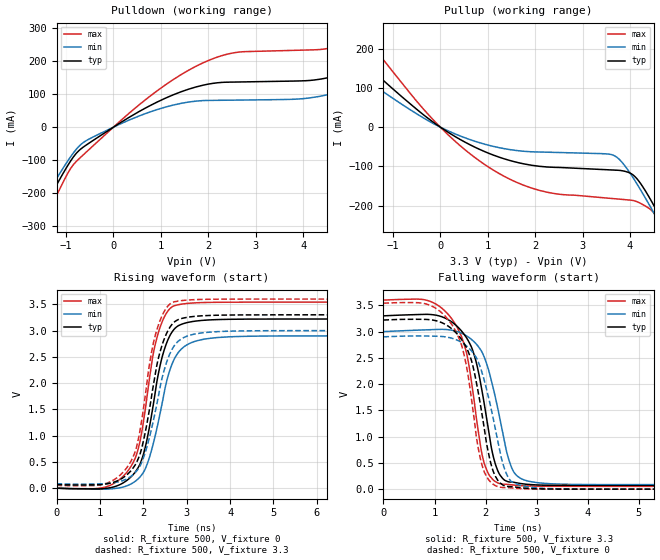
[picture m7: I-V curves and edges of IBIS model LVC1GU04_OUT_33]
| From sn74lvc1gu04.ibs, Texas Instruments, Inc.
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[Model]   LVC1GU04_OUT_33
Model_type  Output
Vref =   0
Rref =   500
Cref =   50p
Vmeas =   1.5
| variable   typ   min   max
C_comp   9.10pF   3.59pF   13.65pF
| C_pullup   10.22pF   4.97pF   13.65pF
| C_pulldown   7.97pF   3.59pF   12.43pF
[Temperature Range]   40   100   -40
| Ambient temperature   25   85   -40
[Voltage range]   3.3   3   3.6
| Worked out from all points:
|   slope of the pulldown table from 0 to 0.495 V, typ, clamps not added: 11.3 ohm
|   slope of the pullup table from 0 to 0.495 V, typ, clamps not added: 13.6 ohm
|   rising waveform, R_fixture 500, V_fixture 0: 20-80 % time 459ps typ, 504ps min, 436ps max; typ from 0 V to 3.22 V
|   falling waveform, R_fixture 500, V_fixture 3.3: 20-80 % time 386ps typ, 413ps min, 377ps max; typ from 3.3 V to 0.069 V
|   rising waveform, R_fixture 500, V_fixture 3.3: 20-80 % time 460ps typ, 505ps min, 433ps max; typ from 0.069 V to 3.3 V
|   falling waveform, R_fixture 500, V_fixture 0: 20-80 % time 389ps typ, 416ps min, 376ps max; typ from 3.22 V to 0 V
[Pulldown]
| LVC1GU04_OUT_33
|   Voltage   I(typ)   I(min)   I(max)
-5.5V     -1.329A    -1.212A    -1.518A
-2.005V   -393.6mA   -353.8mA   -458.1mA
-1.555V   -270.8mA   -242.4mA   -317.5mA
-915mV    -105.6mA   -92.52mA   -128.5mA
-570mV    -54.02mA   -40.71mA   -75.43mA
1.09V     87.67mA    60.7mA     127.9mA
2.375V    136.6mA    81.8mA     220.9mA
4.9V      164.6mA    112.8mA    253.7mA
5.705V    210.7mA    154.2mA    308.6mA
6.855V    302.8mA    233.5mA    425.8mA
7.69V     383.3mA    301.9mA    530.5mA
11V       772.7mA    631.3mA    1.042A
[Pullup]
| LVC1GU04_OUT_33
|   Voltage   I(typ)   I(min)   I(max)
-5.5V     658.4mA    524.1mA    915.7mA
-2.975V   326.7mA    254.3mA    462mA
-2.255V   238.9mA    184.2mA    340.3mA
-1.835V   189.7mA    145.3mA    271.6mA
-90mV     7.531mA    5.5mA      11.13mA
1.035V    -67.22mA   -46.55mA   -103.1mA
2.09V     -99.68mA   -63.32mA   -161mA
3.655V    -109.2mA   -71.84mA   -182mA
4.12V     -127.9mA   -139.4mA   -188.6mA
4.67V     -236.6mA   -254.9mA   -251.4mA
4.83V     -273.4mA   -290.5mA   -289.1mA
11V       -1.848A    -1.769A    -2.022A
[Ramp]
| LVC1GU04_OUT_33
| variable   typ   min   max
dV/dt_r   1.94/4.70E-10   1.75/5.12E-10   2.13/4.44E-10
dV/dt_f   1.96/3.99E-10   1.77/4.29E-10   2.14/3.82E-10
R_load = 500
[Rising Waveform]
| LVC1GU04_OUT_33
R_fixture =   500
C_fixture =   0
L_fixture =   0
V_fixture =   0
V_fixture_min = 0
V_fixture_max = 0
|   Time   V(typ)   V(min)   V(max)
0s        38.55pV    4.76nV     1.659nV
1.19ns    2.758mV    -16.68mV   38.86mV
1.8ns     292.6mV    123.1mV    548.2mV
1.92ns    451.2mV    209.9mV    877.1mV
2.05ns    796.4mV    378.2mV    1.528V
2.22ns    1.54V      818.4mV    2.516V
2.385ns   2.329V     1.417V     3.06V
2.675ns   2.989V     2.388V     3.458V
3.06ns    3.161V     2.753V     3.52V
50ns      3.22V      2.9V       3.541V
[Falling Waveform]
| LVC1GU04_OUT_33
R_fixture =   500
C_fixture =   0
L_fixture =   0
V_fixture =   3.3
V_fixture_min = 3
V_fixture_max = 3.6
|   Time   V(typ)   V(min)   V(max)
0s        3.3V       3V         3.6V
845ps     3.329V     3.034V     3.597V
1.31ns    3.202V     3.031V     3.279V
1.62ns    2.892V     2.923V     2.623V
1.815ns   2.422V     2.765V     1.387V
1.975ns   1.616V     2.51V      486.8mV
2.215ns   409.1mV    1.641V     130.9mV
2.45ns    139.3mV    574.7mV    89.19mV
2.645ns   113.9mV    231.5mV    69.84mV
50ns      69.35mV    85.87mV    53.95mV
[Rising Waveform]
| LVC1GU04_OUT_33
R_fixture =   500
C_fixture =   0
L_fixture =   0
V_fixture =   3.3
V_fixture_min = 3
V_fixture_max = 3.6
|   Time   V(typ)   V(min)   V(max)
0s        69.35mV    85.87mV    53.95mV
1.1ns     75.77mV    84.91mV    80.18mV
1.635ns   264.8mV    184.4mV    406.7mV
1.82ns    452.9mV    301.2mV    713mV
1.955ns   737.6mV    475.1mV    1.251V
2.175ns   1.67V      1.079V     2.52V
2.355ns   2.499V     1.784V     3.124V
2.625ns   3.079V     2.582V     3.513V
2.98ns    3.248V     2.885V     3.579V
50ns      3.3V       3V         3.6V
[Falling Waveform]
| LVC1GU04_OUT_33
R_fixture =   500
C_fixture =   0
L_fixture =   0
V_fixture =   0
V_fixture_min = 0
V_fixture_max = 0
|   Time   V(typ)   V(min)   V(max)
0s        3.22V      2.9V       3.541V
975ps     3.218V     2.913V     3.472V
1.525ns   2.856V     2.797V     2.756V
1.73ns    2.425V     2.626V     1.67V
1.935ns   1.393V     2.203V     439.6mV
2.125ns   410.8mV    1.455V     113mV
2.34ns    78.18mV    480.3mV    31.2mV
2.61ns    36.96mV    97.31mV    15.11mV
3.64ns    825.6uV    3.267mV    163.4uV
50ns      1.802nV    61.14nV    58.11nV
